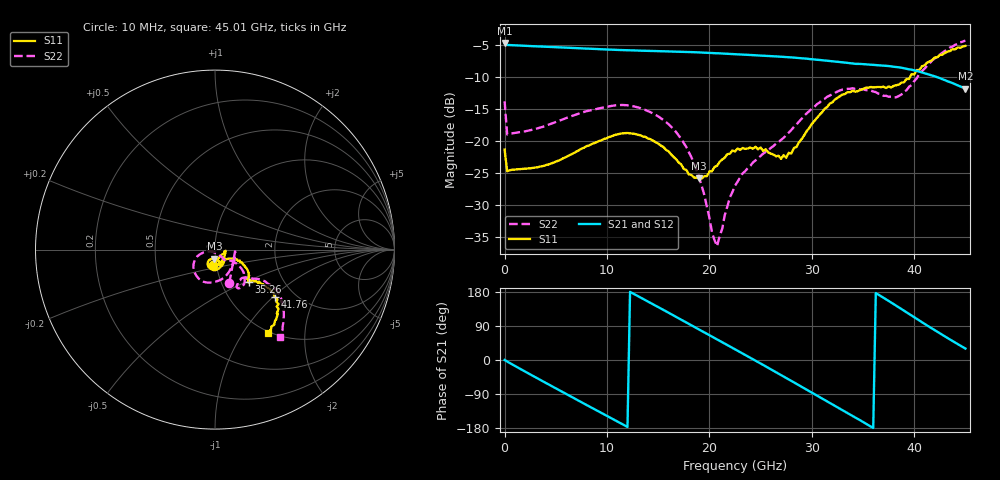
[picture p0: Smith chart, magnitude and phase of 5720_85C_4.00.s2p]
! Device:  ADRF5720
! Description: 0.5dB LSB GaAs MMIC 6-bit Digital Attenuator
! Frequency:  0.000009 -  40 GHz
! Ports:
!	RF1	= Port 1
!	RF2	= Port 2
! Vdd:  3.3 Volt
! Vss:  -3.3 Volt
! Control:  0/3.3 Volt
! State:  4.00 dB attenuation
! Data:  The device was measured using G-S-G Probes on a matrix board.
!  Data was collected using an calibrated 4 port network analyzer.
!  The reference plane for this measurement is at the launchers.
! Note:  Analog Devices supplies this data as a sample of measured data
!  for this product.  Your particular data for this product may vary.
!  Data was taken at 85 degrees C.
!  Analog Devices reserves the right to change this data at anytime.
# GHZ S DB R 45.0
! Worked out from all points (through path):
!   181 points, 10 MHz to 45.01 GHz, reference 45 ohm
!   highest |S21| = -4.74 dB at 10 MHz (marker M1); lowest = -11.9 dB at 45.01 GHz (marker M2)
!   group delay of S21, straight-line fit = 42.2 ps
!   lowest |S11| = -25.9 dB at 19.01 GHz (marker M3), VSWR 1.11, Z = 44.5 - j4.52 ohm
!   |S11| at or under -10 dB: start of sweep to 39.63 GHz
!   |S22| runs from -36.4 to -4.4 dB; largest |S21 - S12| = 0.0029
!   S11 on the Smith chart (normalised r, x): 10 MHz: 0.96, -0.16; 35.26 GHz: 1.35, -0.51; 41.76 GHz: 1.60, -1.03; 45.01 GHz: 0.98, -1.30
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0.01  -21.37 -98.9  -4.74 0.1  -4.73 0.1  -13.85 -66.8
0.26  -24.76 -7.9  -5.06 -4.0  -5.05 -4.0  -19.01 -5.3
2.26  -24.33 -19.2  -5.22 -34.3  -5.20 -34.2  -18.45 -22.9
4.26  -23.73 -37.0  -5.35 -63.8  -5.34 -63.8  -17.53 -44.9
7.76  -21.09 -57.5  -5.61 -115.0  -5.59 -114.9  -15.51 -75.9
11.51  -18.84 -88.4  -5.86 -169.4  -5.85 -169.3  -14.42 -109.0
13.26  -19.13 -103.2  -5.95 165.2  -5.93 165.4  -14.91 -124.9
15.26  -20.75 -116.3  -6.03 136.0  -6.01 136.1  -16.48 -143.2
17.26  -23.70 -117.9  -6.13 106.5  -6.11 106.7  -19.70 -159.6
19.01  -25.88 -93.7  -6.23 80.5  -6.21 80.7  -25.76 -166.9
20.76  -23.90 -73.3  -6.36 54.4  -6.34 54.6  -36.44 -106.5
22.01  -22.03 -68.9  -6.46 35.7  -6.44 35.9  -28.84 -53.4
22.76  -21.20 -70.6  -6.52 24.5  -6.50 24.7  -26.39 -49.8
25.01  -21.05 -72.5  -6.72 -9.3  -6.70 -9.1  -22.38 -47.7
27.51  -22.67 -49.2  -6.95 -47.4  -6.93 -47.1  -19.15 -33.9
30.26  -16.93 -26.0  -7.32 -89.9  -7.30 -89.7  -14.73 -35.9
32.76  -13.04 -33.8  -7.72 -128.6  -7.70 -128.3  -12.15 -48.0
35.26  -11.75 -43.6  -8.08 -167.4  -8.06 -167.1  -12.10 -59.5
37.76  -11.68 -40.1  -8.41 151.7  -8.39 152.1  -13.13 -50.5
39.76  -9.61 -36.5  -8.92 117.3  -8.89 117.7  -11.32 -36.6
41.76  -7.42 -38.3  -9.83 83.0  -9.82 83.5  -7.48 -34.0
45.01  -5.21 -57.6  -11.86 30.3  -11.84 30.6  -4.36 -53.4
